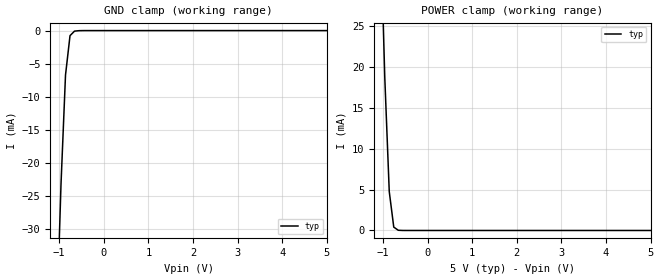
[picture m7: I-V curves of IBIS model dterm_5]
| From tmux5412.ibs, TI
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| dterm_5
[Model]   dterm_5
Model_type   Terminator
|   typ   min   max
C_comp   1.008417e-11   NA   NA
[Voltage Range]   5   NA   NA
[Temperature Range]   27   NA   NA
[Power Clamp Reference]   5   NA   NA
[GND Clamp Reference]   0   NA   NA
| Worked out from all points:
|   GND clamp passes 1 mA (typ) near -0.76 V on its own axis
|   POWER clamp passes 1 mA (typ) near -0.77 V on its own axis
[GND Clamp]
|   Voltage   I(typ)   I(min)   I(max)
-5V       -2.839A    NA         NA
-1.061V   -45mA      NA         NA
-959.6mV  -23.25mA   NA         NA
-858.6mV  -6.731mA   NA         NA
-757.6mV  -768.2uA   NA         NA
-656.6mV  -81.6uA    NA         NA
5V        469.4pA    NA         NA
[POWER Clamp]
|   Voltage   I(typ)   I(min)   I(max)
-5V       2.53A      NA         NA
-1.061V   38.31mA    NA         NA
-959.6mV  18.79mA    NA         NA
-858.6mV  4.751mA    NA         NA
-757.6mV  410.3uA    NA         NA
-656.6mV  26.01uA    NA         NA
5V        -264.5pA   NA         NA
